TYPE LstHeater :
STRUCT
	ToleranceMode:STRING;		//'Value' or 'Percent'
	ToleranceDelayTime:INT;
	WallTemp:INT;
	WallTempWaningRange:INT;
	WallTempAlarmRange:INT;
	
	LidTemp:INT;
	LidTempWaningRange:INT;
	LidTempAlarmRange:INT;
	
	StageEdgeTemp: INT;
	StageEdgeTempWaningRange:INT;
	StageEdgeTempAlarmRange:INT;
	
	StageCenterTemp: INT;
	StageCenterTempWaningRange:INT;
	StageCenterTempAlarmRange:INT;
	
END_STRUCT
END_TYPE
